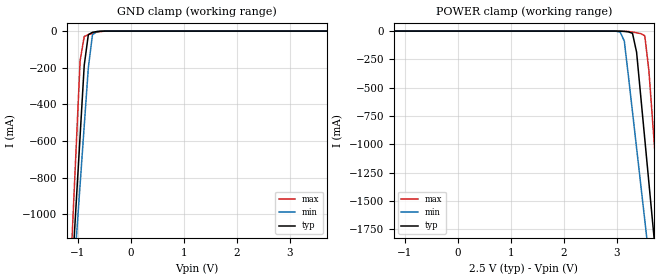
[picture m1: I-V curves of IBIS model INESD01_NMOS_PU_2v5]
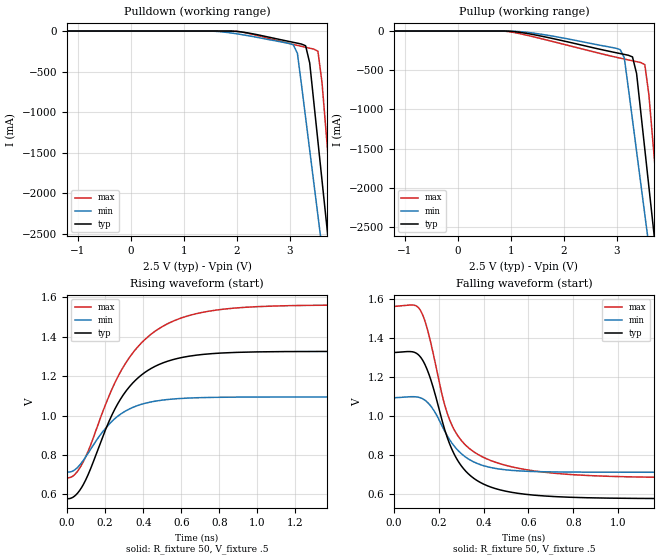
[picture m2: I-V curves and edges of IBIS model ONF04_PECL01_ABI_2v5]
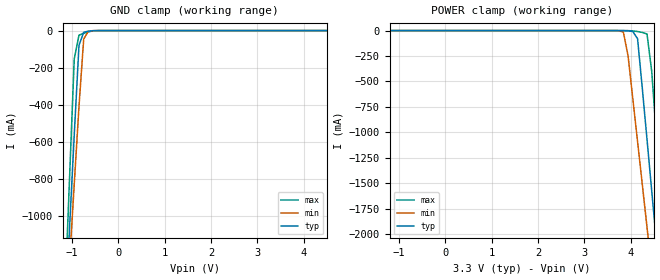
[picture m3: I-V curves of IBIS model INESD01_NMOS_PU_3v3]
|   This file is an IBIS representation of the   |
|   Integrated Devices Technology, Inc.   |
|   ICS843071I   |
|   FEMTOCLOCKS CRYSTAL-TO-3.3V, 2.5V LVPECL CLOCK MULTIPLIER   |
[IBIS Ver]   4.1
[File name]   843081i_01.ibs
[File Rev]   1.0
[Date]   30 Dec 2008 | Last modified
|   24 Dec 2008 | Generated
[Source]   Originated at Integrated Devices Technology, Inc.
[Disclaimer]
IDT hereby grants the user of this IBIS model a non-exclusive,
nontransferable license to use this IBIS model under the following terms.
Before using this IBIS model, the user should read this license.
If the user does not accept these terms,  the IBIS model should be
returned to IDT within 30 days.
   The user is granted this license only to use the IBIS model and
is not granted rights to sell, load, rent, lease or license the IBIS
model in whole or in part, or in modified form to anyone other than
user. User may modify the IBIS model to suit its specific
applications but rights to derivative works and such modifications
shall belong to IDT.
   This IBIS model is provided on an "AS IS" basis and IDT makes
absolutely no warranty with respect to the information contained
herein. IDT DISCLAIMS AND CUSTOMER WAIVES ALL WARRANTIES, EXPRESS
OR IMPLIED, INCLUDING WARRANTIES OF MERCHANTABILITY OR FITNESS FOR
A PARTICULAR PURPOSE. The entire risk as to quality and performance
is with the Customer. ACCORDINGLY, IN NO EVENT SHALL THE COMPANY BE
LIABLE FOR ANY DAMAGES, WHETHER IN CONTRACT OR TORT,INCLUDING ANY
LOST PROFITS OR OTHER INCIDENTAL, CONSEQUENTIAL, EXEMPLARY, OR
PUNITIVE DAMAGES ARISING OUT OF THE USE OR APPLICATION OF THE IBIS
model provided in this package. Further, IDT reserves the right to
make changes without notice to any product herein to improve
reliability, function, or design. IDT does not convey any license
under patent rights or any other intellectual property rights,
including those of third parties.
   IDT is not obligated to provide maintenance or support
for the licensed IBIS model.
[Copyright]   Copyright 2004 byIntegrated Devices Technology, Inc.
[Component]   ICS843081I-01
[Manufacturer] Integrated Devices Technology, Inc.
[Package]
|TSSOP 8 Lead
|   typ   min   max
R_pkg   52.5m   48.8m   56.2m
L_pkg   1.381nH   1.275nH   1.486nH
C_pkg   0.236pF   0.230pF   0.242pF
[Pin]   signal_name   model_name   R_pin   L_pin   C_pin
1   VCC   POWER   56.2m   1.486n   0.242p
2   XTAL_OUT   NC   48.8m   1.275n   0.230p
3   XTAL_IN   NC   48.8m   1.275n   0.230p
4   VEE   GND   56.2m   1.468n   0.242p
5   OE   INESD01_NMOS_PU   56.2m   1.486n   0.242p
6   nQ0   ONF04_PECL01_ABI   48.8m   1.275n   0.230p
7   Q   ONF04_PECL01_ABI   48.8m   1.275n   0.230p
8   VCC   POWER   56.2m   1.468n   0.242p
[Diff Pin]  inv_pin  vdiff tdelay_typ tdelay_min  tdelay_max
7   6   NA   0  0  0
[Model Selector] INESD01_NMOS_PU
INESD01_NMOS_PU_2v5  Buffer selection for 2v5
INESD01_NMOS_PU_3v3  Buffer selection for 3v3
[Model Selector] ONF04_PECL01_ABI
ONF04_PECL01_ABI_2v5  Buffer selection for 2v5
ONF04_PECL01_ABI_3v3  Buffer selection for 3v3
| Models and submodels in the file (4): INESD01_NMOS_PU_2v5 (Input), ONF04_PECL01_ABI_2v5 (Output_ECL), INESD01_NMOS_PU_3v3 (Input), ONF04_PECL01_ABI_3v3 (Output_ECL)
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[Model] INESD01_NMOS_PU_2v5
Model_type   Input
Polarity   Non-Inverting
Vinl = 0.5V
Vinh = 1.1V
|   typ   min   max
C_comp   2pF   1.5pF   2.5pF
|   typ   min   max
[Voltage range]  2.5V   2.375V   2.625V
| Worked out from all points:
|   GND clamp passes 1 mA (typ) near -0.57 V on its own axis
[GND_clamp]
|Voltage I(typ)   I(min)   I(max)
-2.5V     -8.263A    -7.237A    -9.981A
-1.108V   -1.337A    -1.473A    -1.142A
-1.031V   -953.1mA   -1.154A    -651.2mA
-953.6mV  -569.5mA   -835mA     -160.3mA
-876.3mV  -186.2mA   -516.8mA   -29.47mA
-799mV    -19.59mA   -199.2mA   -19.31mA
-721.6mV  -6.713mA   -20.65mA   -12.35mA
-644.3mV  -2.945mA   -2.694mA   -6.489mA
-489.7mV  -219.7uA   -96.65uA   -544uA
5V        555.4pA    974.3pA    139.3pA
[POWER_clamp]
|Voltage   I(typ)   I(min)   I(max)
-2.5V     555.4pA    852.5pA    162.9pA
3.067V    -971.3uA   -8.981mA   -175.9uA
3.144V    -2.945mA   -87.2mA    -1.018mA
3.299V    -19.59mA   -713mA     -8.571mA
3.376V    -186.2mA   -1.031A    -14.91mA
3.454V    -569.5mA   -1.35A     -22.33mA
3.531V    -953.1mA   -1.669A    -41.51mA
3.608V    -1.337A    -1.989A    -348.5mA
3.686V    -1.721A    -2.309A    -839.4mA
3.763V    -2.106A    -2.628A    -1.33A
3.84V     -2.49A     -2.948A    -1.822A
5V        -8.263A    -7.755A    -9.188A
[Model] ONF04_PECL01_ABI_2v5
Model_type  Output_ECL
Polarity   Non-Inverting
Vmeas = .975
Rref = 50
Cref = 0
Vref = .5
|Variable  typ   min   max
C_comp   2p   1.5p   2.5p
[Voltage Range]   2.5   2.375   2.625
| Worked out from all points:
|   rising waveform, R_fixture 50, V_fixture .5: 20-80 % time 234ps typ, 201ps min, 282ps max; typ from 0.578 V to 1.33 V
|   falling waveform, R_fixture 50, V_fixture .5: 20-80 % time 146ps typ, 137ps min, 151ps max; typ from 1.33 V to 0.578 V
| Open source, no load
|  Voltage   I(typ)   I(min)   I(max)
[Pullup]
-2.5V     0A         1.541pA    0A
902.1mV   -652.8uA   -160uA     -3.042mA
3.067V    -287.8mA   -237.7mA   -346mA
3.144V    -298.5mA   -342mA     -357.6mA
3.299V    -330.4mA   -1.134A    -380.1mA
3.376V    -542.4mA   -1.536A    -391.2mA
3.531V    -1.506A    -2.34A     -427.9mA
3.608V    -1.988A    -2.742A    -812.5mA
3.686V    -2.47A     -3.144A    -1.427A
3.763V    -2.952A    -3.545A    -2.041A
3.84V     -3.434A    -3.947A    -2.655A
5V        -10.66A    -9.976A    -11.86A
[Pulldown]
-2.5V     0A         1.541pA    0A
1.907V    -1.197mA   -25.19mA   -528.7uA
3.067V    -139.2mA   -170.1mA   -165.3mA
3.144V    -149.7mA   -274mA     -177.1mA
3.299V    -181.3mA   -1.066A    -200.1mA
3.376V    -393.2mA   -1.467A    -211.4mA
3.454V    -875mA     -1.869A    -222.9mA
3.531V    -1.357A    -2.271A    -248.5mA
3.608V    -1.839A    -2.672A    -633.4mA
3.686V    -2.321A    -3.074A    -1.248A
3.84V     -3.284A    -3.878A    -2.476A
5V        -10.51A    -9.903A    -11.69A
[Ramp]
|   typ   min   max
dV/dt_r   0.598/0.377n   0.305/0.319n   0.702/0.456n
dV/dt_f   0.602/0.256n   0.309/0.228n   0.707/0.292n
R_load =   50.0000
[Rising Waveform]
R_fixture = 50
V_fixture = .5   | VCC_typ - 2V
V_fixture_max = 0.625   | VCC_max - 2V
V_fixture_min = 0.375   | VCC_min - 2V
C_fixture = 0.0p
| Time   typ   min   max
0s        578.1mV    713.3mV    684.3mV
42ps      593.1mV    725.4mV    702.3mV
86.1ps    651mV      773.6mV    767.4mV
228.9ps   988.8mV    964mV      1.119V
310.8ps   1.126V     1.025V     1.271V
417.9ps   1.225V     1.064V     1.394V
548.1ps   1.282V     1.083V     1.475V
714ps     1.31V      1.091V     1.524V
942.9ps   1.322V     1.094V     1.55V
1.999ns   1.326V     1.094V     1.562V
[Falling Waveform]
R_fixture = 50
V_fixture = .5   | VCC_typ - 2V
V_fixture_max = 0.625   | VCC_max - 2V
V_fixture_min = 0.375   | VCC_min - 2V
C_fixture = 0.0p
| Time   typ   min   max
0s        1.326V     1.094V     1.562V
88.2ps    1.328V     1.1V       1.568V
117.6ps   1.304V     1.094V     1.542V
159.6ps   1.203V     1.059V     1.398V
220.5ps   954.3mV    936.4mV    1.083V
260.4ps   825.8mV    859.8mV    949.9mV
331.8ps   705.4mV    781.5mV    839.2mV
434.7ps   636.4mV    736.8mV    772mV
856.8ps   583mV      713.7mV    697.1mV
1.999ns   578mV      713.3mV    684.3mV
[Model] INESD01_NMOS_PU_3v3
Model_type   Input
Polarity   Non-Inverting
Vinl = 0.7V
Vinh = 1.3V
|   typ   min   max
C_comp   2pF   1.5pF   2.5pF
|   typ   min   max
[Voltage range]  3.3V   3.15V   3.45V
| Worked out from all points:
|   GND clamp passes 1 mA (typ) near -0.56 V on its own axis
[GND_clamp]
|Voltage   I(typ)   I(min)   I(max)
-3.3V     -12.24A    -10.56A    -15.06A
-1.157V   -1.578A    -1.673A    -1.45A
-1.055V   -1.071A    -1.251A    -801.8mA
-952.6mV  -564.4mA   -830.8mA   -154mA
-850.5mV  -79.92mA   -410.9mA   -24.97mA
-748.5mV  -8.956mA   -45.87mA   -14.66mA
-646.4mV  -3.019mA   -2.828mA   -6.626mA
-544.3mV  -652uA     -309.6uA   -1.636mA
6.6V      4.435nA    6.865nA    1.283nA
[POWER_clamp]
|Voltage   I(typ)   I(min)   I(max)
-3.3V     4.435nA    5.64nA     1.609nA
3.64V     -5.052uA   -135.1uA   -13.25nA
3.844V    -652uA     -14.51mA   -32.02uA
3.946V    -3.019mA   -250.2mA   -451.4uA
4.048V    -8.956mA   -669.7mA   -3.083mA
4.151V    -79.92mA   -1.09A     -9.442mA
4.355V    -1.071A    -1.933A    -33.35mA
4.457V    -1.578A    -2.355A    -402.1mA
4.559V    -2.085A    -2.777A    -1.05A
4.661V    -2.593A    -3.199A    -1.698A
4.763V    -3.101A    -3.622A    -2.347A
6.6V      -12.24A    -11.24A    -14.01A
